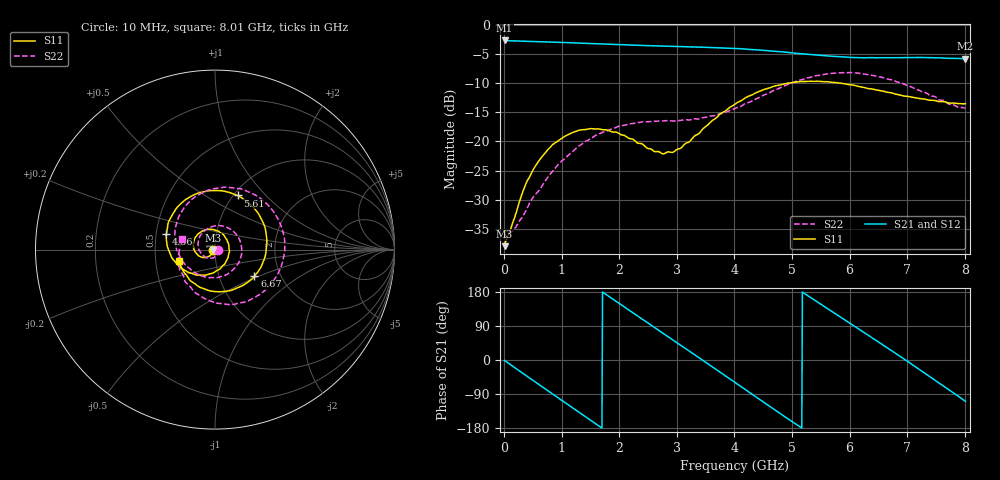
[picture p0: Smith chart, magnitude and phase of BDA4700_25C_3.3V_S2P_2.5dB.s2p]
!Agilent Technologies,E5071B,MY42404982,A.09.10
!Date: Mon Oct 20 18:04:01 2025
!Data & Calibration Information:
!Freq	S11:SOLT2(ON)	S21:SOLT2(ON)	S12:SOLT2(ON)	S22:SOLT2(ON)
# Hz S RI R 50
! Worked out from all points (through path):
!   801 points, 10 MHz to 8.01 GHz, reference 50 ohm
!   highest |S21| = -2.61 dB at 10 MHz (marker M1); lowest = -5.8 dB at 8.01 GHz (marker M2)
!   group delay of S21, straight-line fit = 286 ps
!   lowest |S11| = -38.0 dB at 10 MHz (marker M3), VSWR 1.03, Z = 48.8 - j0.174 ohm
!   |S11| at or under -10 dB: start of sweep to 4.902 GHz; 5.862 GHz to end of sweep
!   |S22| runs from -36.4 to -8.1 dB; largest |S21 - S12| = 0.0083
!   S11 on the Smith chart (normalised r, x): 10 MHz: 0.98, -0.00; 4.56 GHz: 0.57, +0.11; 5.61 GHz: 1.05, +0.71; 6.67 GHz: 1.47, -0.47; 8.01 GHz: 0.66, -0.09
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1e7  -0.0124 -0.00179  0.74 -0.0158  0.7396 -0.0165  0.0162 -0.00152
3.3e8  -0.0232 -0.0294  0.5933 -0.4231  0.5929 -0.4233  0.0172 -0.0151
7.1e8  -0.0662 -0.0438  0.1774 -0.697  0.1776 -0.6971  -0.00672 -0.0448
1.02e9  -0.1063 -0.0189  -0.2237 -0.6744  -0.2238 -0.6746  -0.055 -0.0415
1.35e9  -0.1204 0.0364  -0.5601 -0.4216  -0.5602 -0.422  -0.0933 0.0166
1.63e9  -0.0961 0.085  -0.6865 -0.0926  -0.6867 -0.0924  -0.0771 0.0854
1.92e9  -0.0447 0.1121  -0.6311 0.2624  -0.6316 0.2624  -0.00537 0.1308
2.32e9  0.0338 0.0906  -0.2953 0.6038  -0.2952 0.6039  0.1114 0.093
2.68e9  0.0763 0.029  0.1282 0.6515  0.1272 0.6514  0.1485 -0.0209
3.36e9  0.017 -0.1137  0.6417 0.0966  0.6423 0.0962  -0.00661 -0.1559
3.67e9  -0.069 -0.1416  0.587 -0.2575  0.5868 -0.2592  -0.1009 -0.1337
4.01e9  -0.1789 -0.1098  0.3222 -0.5431  0.3234 -0.5421  -0.181 -0.0646
4.56e9  -0.2711 0.0869  -0.2734 -0.54  -0.2726 -0.5409  -0.2162 0.1369
4.97e9  -0.186 0.26  -0.543 -0.2056  -0.5436 -0.2076  -0.103 0.2984
5.35e9  -0.00797 0.3292  -0.5311 0.1735  -0.5322 0.1703  0.1061 0.3431
5.61e9  0.1262 0.3015  -0.3913 0.3786  -0.392 0.379  0.254 0.2843
6.12e9  0.283 0.101  0.0416 0.5254  0.0456 0.526  0.3888 -0.00276
6.67e9  0.2193 -0.1485  0.4529 0.2664  0.4531 0.2653  0.21 -0.2715
6.68e9  0.2161 -0.1522  0.4573 0.2584  0.4584 0.2575  0.2054 -0.2744
7.25e9  -0.00725 -0.2332  0.4613 -0.2562  0.4607 -0.2566  -0.0871 -0.2548
7.64e9  -0.1391 -0.171  0.1791 -0.4895  0.1789 -0.4901  -0.1979 -0.1078
8.01e9  -0.2021 -0.0619  -0.167 -0.4871  -0.1654 -0.4879  -0.1853 0.0572
